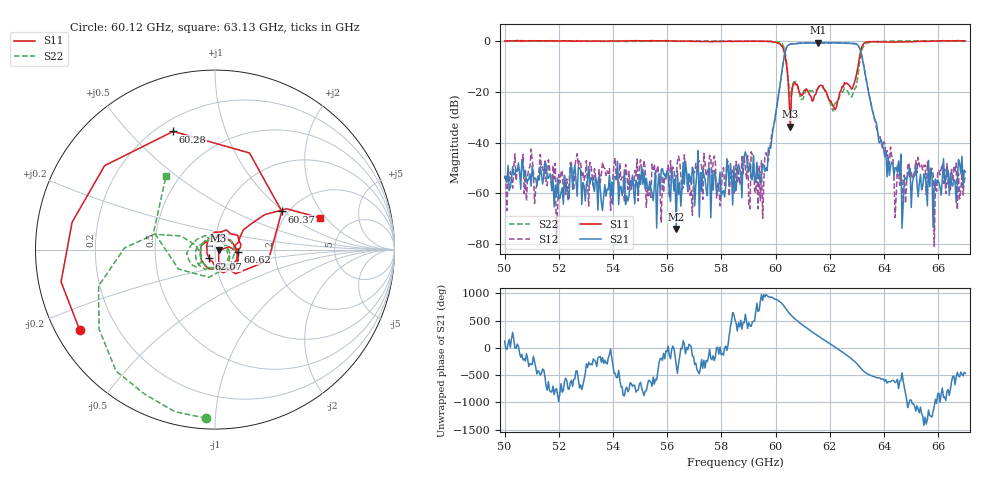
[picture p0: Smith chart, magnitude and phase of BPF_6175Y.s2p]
!Agilent Technologies,E8361A,US42410132,A.06.03.05
!Agilent E8361A: A.06.03.05
!Date: Friday, July 11, 2008 14:50:20
!Correction: S11(Full 2 Port(1,2)) S21(Full 2 Port(1,2)) S12(Full 2 Port(1,2)) S22(Full 2 Port(1,2))
!S2P File: Measurements: S11, S21, S12, S22:
# Hz S  MA  R 50
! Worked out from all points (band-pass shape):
!   401 points, 50 GHz to 67 GHz, reference 50 ohm
!   highest |S21| = -0.74 dB at 61.56 GHz (marker M1); lowest = -73.9 dB at 56.33 GHz (marker M2)
!   |S21| within 3 dB of the highest: 60.37 GHz to 63.13 GHz (2.758 GHz wide, 4.47 % of centre)
!   lowest |S11| = -33.8 dB at 60.54 GHz (marker M3), VSWR 1.04, Z = 52 - j0.513 ohm
!   |S11| at or under -10 dB: 60.41 GHz to 63.04 GHz (2.631 GHz wide, 4.26 % of centre)
!   |S22| runs from -27.6 to 0.1 dB; largest |S21 - S12| = 0.025
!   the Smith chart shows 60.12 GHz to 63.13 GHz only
!   S11 on the Smith chart (normalised r, x): 60.12 GHz: 0.07, -0.28; 60.28 GHz: 0.26, +0.67; 60.37 GHz: 1.86, +0.97; 60.62 GHz: 1.29, -0.03; 62.07 GHz: 0.93, -0.09; 63.13 GHz: 3.07, +1.73
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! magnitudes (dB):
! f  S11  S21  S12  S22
! 50 GHz  -0.2  -54.0  -53.0  -0.1
! 52.85 GHz  -0.1  -64.4  -52.9  -0.1
! 55.7 GHz  -0.1  -52.1  -53.9  -0.1
! 56.33 GHz  -0.2  -73.9  -53.2  -0.2
! 56.84 GHz  -0.2  -53.5  -60.8  -0.1
! 57.14 GHz  -0.3  -43.2  -46.9  -0.1
! 58.5 GHz  -0.2  -59.0  -58.4  -0.2
! 58.88 GHz  0.0  -43.7  -49.7  -0.3
! 59.44 GHz  -0.1  -56.0  -62.8  -0.2
! 60.12 GHz  -1.1  -21.0  -20.9  -0.5
! 60.28 GHz  -3.1  -8.2  -8.1  -2.1
! 60.37 GHz  -7.4  -3.7  -3.6  -5.9
! 60.54 GHz  -33.8  -1.4  -1.4  -21.7
! 60.62 GHz  -18.0  -1.3  -1.2  -16.9
! 61.35 GHz  -23.7  -0.9  -0.8  -19.8
! 61.56 GHz  -18.5  -0.7  -0.8  -19.0
! 62.07 GHz  -24.5  -0.8  -0.8  -26.4
! 63.13 GHz  -4.3  -3.9  -3.8  -6.1
! 64.19 GHz  -0.6  -52.9  -48.5  -0.1
! 64.49 GHz  -0.4  -51.7  -48.5  -0.1
! 64.75 GHz  -0.5  -54.7  -52.7  0.0
! 67 GHz  -0.1  -51.5  -53.3  -0.2
